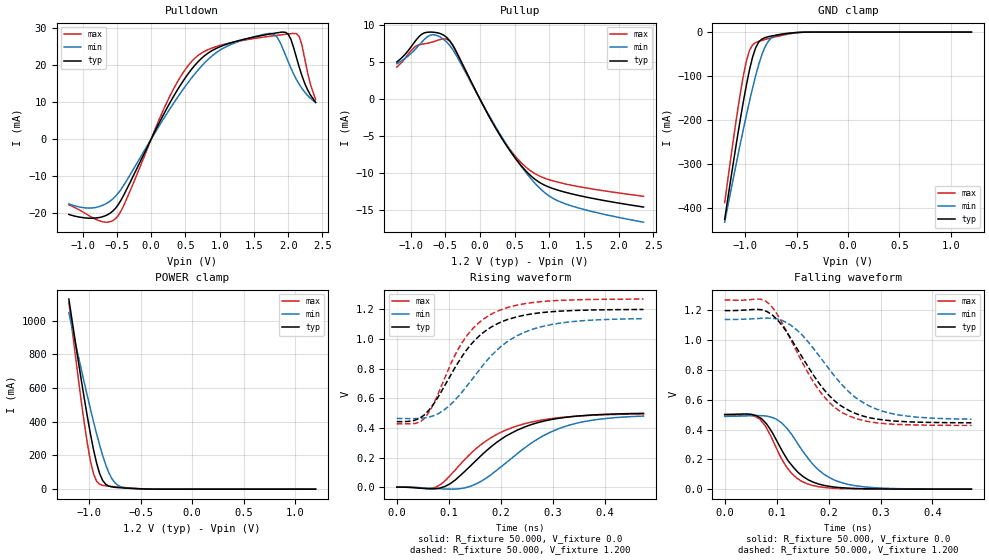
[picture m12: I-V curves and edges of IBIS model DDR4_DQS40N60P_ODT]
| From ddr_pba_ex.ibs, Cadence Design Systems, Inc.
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|   Model DDR4_DQS40N60P_ODT
[Model]   DDR4_DQS40N60P_ODT
Model_type I/O
Polarity   Non-Inverting
Enable   Active-High
Vinl =  0.823V
Vinh =  0.887V
C_comp   1.720pF   1.734pF   1.730pF
C_comp_pullup   0.538pF   0.595pF   0.526pF
C_comp_pulldown   1.182pF   1.139pF   1.204pF
[Model Spec]
Vinh   0.887V   NA   NA
Vinl   0.823V   NA   NA
Vmeas   0.840V   NA   NA
[Add Submodel]
|  Submodel_name   Mode
DDR4_DQS_ODT60   Non-Driving
[Temperature Range]   27.000   0.125k   -40.000
[Voltage Range]   1.200V   1.140V   1.270V
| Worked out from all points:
|   slope of the pulldown table from 0 to 0.18 V, typ, clamps not added: 27.2 ohm
|   slope of the pullup table from 0 to 0.18 V, typ, clamps not added: 57.4 ohm
|   GND clamp passes 1 mA (typ) near -0.50 V on its own axis
|   POWER clamp passes 1 mA (typ) near -0.46 V on its own axis
|   rising waveform, R_fixture 50.000, V_fixture 0.0: 20-80 % time 112ps typ, 118ps min, 109ps max; typ from 0.001 V to 0.499 V
|   rising waveform, R_fixture 50.000, V_fixture 1.200: 20-80 % time 91.2ps typ, 107ps min, 79.9ps max; typ from 0.443 V to 1.2 V
|   falling waveform, R_fixture 50.000, V_fixture 0.0: 20-80 % time 57.6ps typ, 68.4ps min, 48.5ps max; typ from 0.502 V to 0 V
|   falling waveform, R_fixture 50.000, V_fixture 1.200: 20-80 % time 89.7ps typ, 100ps min, 84.4ps max; typ from 1.2 V to 0.446 V
[Pulldown]
|Voltage   I(typ)   I(min)   I(max)
-1.2V     -20.33mA   -17.47mA   -17.73mA
-840mV    -21.33mA   -18.52mA   -21.33mA
-520mV    -18.67mA   -15.43mA   -21.47mA
400mV     13.8mA     11.7mA     16mA
640mV     20.01mA    17.69mA    21.92mA
960mV     24.62mA    23.51mA    25.09mA
1.76V     28.51mA    28.56mA    27.88mA
1.84V     28.75mA    27.53mA    28.07mA
2V        28.39mA    20.97mA    28.43mA
2.12V     22.12mA    16.15mA    28.51mA
2.2V      17.21mA    13.75mA    25.48mA
2.4V      9.967mA    9.905mA    10.69mA
[Pullup]
|Voltage   I(typ)   I(min)   I(max)
-1.2V     5.02mA     4.773mA    4.338mA
-960mV    7.514mA    6.485mA    6.876mA
-840mV    8.783mA    7.706mA    7.425mA
-720mV    9.066mA    8.641mA    7.63mA
-560mV    8.818mA    8.321mA    8.099mA
-400mV    7.394mA    6.807mA    7.432mA
280mV     -4.745mA   -4.576mA   -4.71mA
520mV     -8.111mA   -8.075mA   -7.827mA
760mV     -10.57mA   -11.01mA   -9.882mA
960mV     -11.75mA   -12.82mA   -10.77mA
1.2V      -12.51mA   -14.04mA   -11.39mA
2.36V     -14.59mA   -16.63mA   -13.13mA
[GND_clamp]
|Voltage   I(typ)   I(min)   I(max)
-1.2V     -426.2mA   -432.8mA   -388.3mA
-1.08V    -244.1mA   -290.9mA   -187.6mA
-1.02V    -160.2mA   -222.9mA   -101.2mA
-990mV    -121.8mA   -190.1mA   -66.76mA
-960mV    -87.12mA   -158.5mA   -42.47mA
-900mV    -36.37mA   -100.2mA   -23.99mA
-840mV    -16.17mA   -52.6mA    -18.98mA
-810mV    -12.75mA   -34.94mA   -17.06mA
-750mV    -9.219mA   -14.09mA   -13.42mA
-600mV    -3.476mA   -2.979mA   -5.372mA
-390mV    -77.95uA   -145.6uA   -88.64uA
1.2V      1.562nA    185.8nA    255.1pA
[POWER_clamp]
|Voltage   I(typ)   I(min)   I(max)
-1.2V     1.129A     1.047A     1.109A
-1.08V    651.1mA    713.3mA    524.8mA
-1.02V    430.1mA    553.1mA    270.8mA
-990mV    328mA      475.7mA    167mA
-960mV    234.7mA    400.6mA    90.32mA
-930mV    154.2mA    328.7mA    47.17mA
-900mV    91.53mA    260.8mA    29.3mA
-840mV    28.2mA     142.5mA    19.67mA
-780mV    13.3mA     60.49mA    15.94mA
-720mV    9.309mA    21.57mA    12.7mA
-660mV    6.902mA    8.818mA    9.642mA
1.2V      -4.11nA    -153.5nA   -871.8pA
[Ramp]
| variable   typ   min   max
dV/dt_r 0.301/0.116n   0.289/0.124n   0.299/0.114n
dV/dt_f 0.453/95.262p   0.403/0.105n   0.505/86.557p
R_load = 50.000
| The next line is not an IBIS keyword
| [Initial Delay]   0.325ns   0.500ns   0.200ns
[Rising Waveform]
R_fixture= 50.000
V_fixture= 0.0
V_fixture_min= 0.0
V_fixture_max= 0.0
|time   V(typ)   V(min)   V(max)
0s        1.431mV    990.4uV    403.8uV
65ps      -10.3mV    -6.386mV   -7.604mV
92ps      4.496mV    -11.39mV   41.65mV
129ps     101.2mV    -5.303mV   180.8mV
159ps     203.3mV    33.55mV    279.5mV
200ps     322.4mV    135.9mV    370.2mV
235ps     390.4mV    235.6mV    417.5mV
280ps     444mV      343.9mV    454mV
330ps     474mV      417mV      475.6mV
475ps     498.7mV    480.4mV    494.7mV
[Rising Waveform]
R_fixture= 50.000
V_fixture= 1.200
V_fixture_min= 1.140
V_fixture_max= 1.270
|time   V(typ)   V(min)   V(max)
0s        443.2mV    464.6mV    427.8mV
36ps      454.5mV    463.4mV    431mV
55ps      495.1mV    469.3mV    471.8mV
89ps      664.8mV    517mV      709.9mV
126ps     884.2mV    643.6mV    977.4mV
155ps     1.008V     773.4mV    1.1V
186ps     1.089V     902.2mV    1.175V
229ps     1.147V     1.017V     1.227V
280ps     1.178V     1.085V     1.253V
475ps     1.199V     1.137V     1.269V
[Falling Waveform]
R_fixture= 50.000
V_fixture= 0.0
V_fixture_min= 0.0
V_fixture_max= 0.0
|time   V(typ)   V(min)   V(max)
0s        501.6mV    488.5mV    497.6mV
48ps      503.7mV    493.7mV    497.2mV
67ps      481.4mV    494.2mV    471.4mV
78ps      447.8mV    491.9mV    426.5mV
99ps      333.5mV    470.9mV    278.5mV
128ps     164.7mV    371.9mV    109.3mV
167ps     52.55mV    178.3mV    26.75mV
200ps     19.49mV    80.66mV    8.46mV
249ps     5.068mV    24.42mV    1.852mV
475ps     117.5uV    212.5uV    51.07uV
[Falling Waveform]
R_fixture= 50.000
V_fixture= 1.200
V_fixture_min= 1.140
V_fixture_max= 1.270
|time   V(typ)   V(min)   V(max)
0s        1.199V     1.139V     1.27V
67ps      1.206V     1.147V     1.276V
87ps      1.18V      1.149V     1.24V
111ps     1.098V     1.132V     1.114V
140ps     939.8mV    1.066V     914.2mV
187ps     687mV      871.2mV    638.8mV
228ps     550.9mV    692.4mV    510.4mV
269ps     488.4mV    575.9mV    459.2mV
310ps     462.8mV    517.3mV    439.5mV
475ps     445.6mV    469.7mV    428.1mV
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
